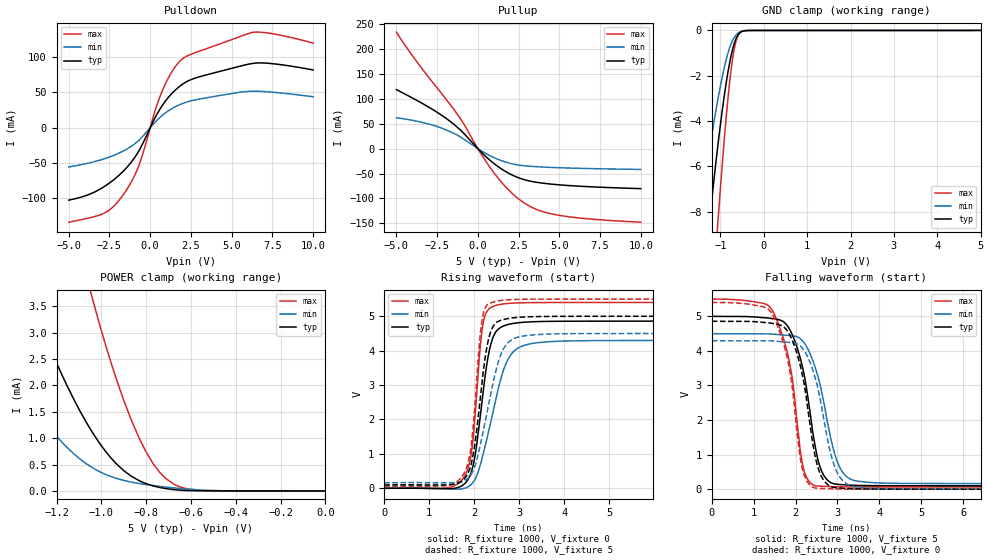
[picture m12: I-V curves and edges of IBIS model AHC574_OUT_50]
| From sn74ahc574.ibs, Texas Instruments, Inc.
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[Model]   AHC574_OUT_50
Model_type  3-state
Enable   Active-Low
Vref =   0
Rref =   1000
Cref =   50p
Vmeas =   2.5
| variable   typ   min   max
C_comp   1.98pF   1.73pF   2.11pF
| C_pullup   3.11pF   1.84pF   3.96pF
| C_pulldown   2.29pF   1.73pF   2.86pF
| C_tri-state   1.98pF   1.73pF   2.11pF
[Temperature Range]   40   100   -40
| Ambient temperature   25   85   -40
[Voltage range]   5   4.5   5.5
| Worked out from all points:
|   slope of the pulldown table from 0 to 0.75 V, typ, clamps not added: 23.5 ohm
|   slope of the pullup table from 0 to 0.75 V, typ, clamps not added: 32 ohm
|   GND clamp passes 1 mA (typ) near -0.74 V on its own axis
|   POWER clamp passes 1 mA (typ) near -1.02 V on its own axis
|   rising waveform, R_fixture 1000, V_fixture 0: 20-80 % time 295ps typ, 478ps min, 208ps max; typ from 0 V to 4.86 V
|   falling waveform, R_fixture 1000, V_fixture 5: 20-80 % time 436ps typ, 494ps min, 414ps max; typ from 5 V to 0.098 V
|   rising waveform, R_fixture 1000, V_fixture 5: 20-80 % time 282ps typ, 432ps min, 206ps max; typ from 0.098 V to 5 V
|   falling waveform, R_fixture 1000, V_fixture 0: 20-80 % time 422ps typ, 464ps min, 407ps max; typ from 4.86 V to 0 V
[GND Clamp]
| AHC574_OUT_50
|   Voltage   I(typ)   I(min)   I(max)
-5V       -113.3mA   -74.38mA   -144.1mA
-1.5V     -13.41mA   -8.512mA   -21.28mA
-1.27V    -8.779mA   -5.481mA   -14.35mA
-1.245V   -8.31mA    -5.173mA   -13.62mA
-1.07V    -5.247mA   -3.165mA   -8.756mA
-1.05V    -4.925mA   -2.954mA   -8.229mA
-875mV    -2.411mA   -1.348mA   -3.999mA
-765mV    -1.211mA   -644.1uA   -1.902mA
-665mV    -482.4uA   -260.9uA   -658.7uA
-615mV    -260.9uA   -150.8uA   -320uA
-545mV    -91.06uA   -60.8uA    -92.76uA
5V        41.61nA    4.676uA    381.8nA
[POWER Clamp]
| AHC574_OUT_50
|   Voltage   I(typ)   I(min)   I(max)
-5V       92.48mA    58.78mA    149.9mA
-1.605V   7.347mA    3.826mA    15.8mA
-1.575V   6.917mA    3.572mA    15.03mA
-1.325V   3.729mA    1.737mA    9.054mA
-1.175V   2.193mA    921.2uA    5.995mA
-1.065V   1.285mA    509.1uA    4.052mA
-1.04V    1.11mA     440.1uA    3.651mA
-935mV    523.3uA    240.6uA    2.146mA
-830mV    191.8uA    139.8uA    989.8uA
-710mV    43.14uA    72.34uA    227.2uA
-545mV    1.272uA    12.21uA    8.176uA
-84.45fV  41.61nA    2.414nA    581.8nA
[Pulldown]
| AHC574_OUT_50
|   Voltage   I(typ)   I(min)   I(max)
-5V       -102.6mA   -55.6mA    -133.8mA
-2.78V    -82.71mA   -43.68mA   -120.5mA
-2.225V   -73.44mA   -39.02mA   -110.8mA
-1.61V    -60.55mA   -32.45mA   -93.44mA
-700mV    -32.97mA   -17.85mA   -53.73mA
310mV     14.74mA    8.08mA     24.97mA
795mV     33.37mA    18.5mA     55.24mA
1.41V     50.51mA    28.16mA    82.14mA
2V        61.97mA    34.49mA    98mA
3.01V     72.15mA    40.66mA    108.5mA
6.35V     91.3mA     51.8mA     135.3mA
10V       81.91mA    43.96mA    119.9mA
[Pullup]
| AHC574_OUT_50
|   Voltage   I(typ)   I(min)   I(max)
-5V       118.3mA    61.85mA    233.6mA
-3.725V   96.33mA    54.83mA    173.3mA
-1.74V    55.61mA    34.63mA    90.14mA
-930mV    32.84mA    20.44mA    53.02mA
125mV     -4.276mA   -2.671mA   -6.772mA
890mV     -27.29mA   -16.57mA   -44.24mA
1.705V    -45.94mA   -26.95mA   -76.63mA
2.52V     -58.72mA   -33.01mA   -101.2mA
3.53V     -67.14mA   -36.14mA   -121mA
4.76V     -71.97mA   -38.08mA   -132.4mA
6.77V     -76.3mA    -39.95mA   -140.8mA
10V       -80.28mA   -41.8mA    -147.5mA
[Ramp]
| AHC574_OUT_50
| variable   typ   min   max
dV/dt_r   2.92/2.98E-10   2.59/4.84E-10   3.24/2.11E-10
dV/dt_f   2.94/4.39E-10   2.60/4.98E-10   3.26/4.15E-10
R_load = 1000
[Rising Waveform]
| AHC574_OUT_50
R_fixture =   1000
C_fixture =   0
L_fixture =   0
V_fixture =   0
V_fixture_min = 0
V_fixture_max = 0
|   Time   V(typ)   V(min)   V(max)
0s        858.1pV    1.441nV    521.7pV
1.765ns   109.5mV    -6.706mV   308mV
1.955ns   559.9mV    143.3mV    1.21V
2.135ns   2.1V       677.9mV    4.131V
2.215ns   2.986V     1.081V     4.906V
2.42ns    4.393V     2.23V      5.288V
2.765ns   4.765V     3.782V     5.375V
3.21ns    4.835V     4.189V     5.396V
4.515ns   4.857V     4.291V     5.401V
50ns      4.858V     4.296V     5.401V
[Falling Waveform]
| AHC574_OUT_50
R_fixture =   1000
C_fixture =   0
L_fixture =   0
V_fixture =   5
V_fixture_min = 4.5
V_fixture_max = 5.5
|   Time   V(typ)   V(min)   V(max)
0s        5V         4.5V       5.5V
1.455ns   4.933V     4.486V     5.149V
1.82ns    4.7V       4.449V     3.874V
2.035ns   4.109V     4.409V     1.979V
2.205ns   3.317V     4.237V     531mV
2.49ns    1.106V     3.445V     97.07mV
2.71ns    336.5mV    2.289V     79.2mV
3.065ns   134.1mV    610.6mV    68.55mV
3.86ns    102.5mV    188.5mV    63.59mV
50ns      97.66mV    160.9mV    62.46mV
[Rising Waveform]
| AHC574_OUT_50
R_fixture =   1000
C_fixture =   0
L_fixture =   0
V_fixture =   5
V_fixture_min = 4.5
V_fixture_max = 5.5
|   Time   V(typ)   V(min)   V(max)
0s        97.66mV    160.9mV    62.46mV
1.36ns    98.88mV    162.2mV    76.32mV
1.745ns   230.4mV    199.6mV    368.9mV
1.93ns    686.6mV    400.5mV    1.213V
2.12ns    2.439V     1.177V     4.276V
2.205ns   3.432V     1.697V     5.091V
2.39ns    4.63V      2.885V     5.402V
2.7ns     4.921V     4.156V     5.474V
4.345ns   4.999V     4.497V     5.5V
50ns      5V         4.5V       5.5V
[Falling Waveform]
| AHC574_OUT_50
R_fixture =   1000
C_fixture =   0
L_fixture =   0
V_fixture =   0
V_fixture_min = 0
V_fixture_max = 0
|   Time   V(typ)   V(min)   V(max)
0s        4.858V     4.296V     5.401V
1.45ns    4.795V     4.288V     5.052V
1.815ns   4.557V     4.25V      3.732V
2.02ns    3.982V     4.21V      1.81V
2.19ns    3.146V     4.04V      466.2mV
2.49ns    836.3mV    3.128V     31.65mV
2.69ns    228.9mV    1.927V     16.53mV
3ns       36.84mV    468.1mV    6.755mV
3.795ns   4.923mV    26.91mV    1.277mV
50ns      -43.66pV   -1.289nV   87.28pV
